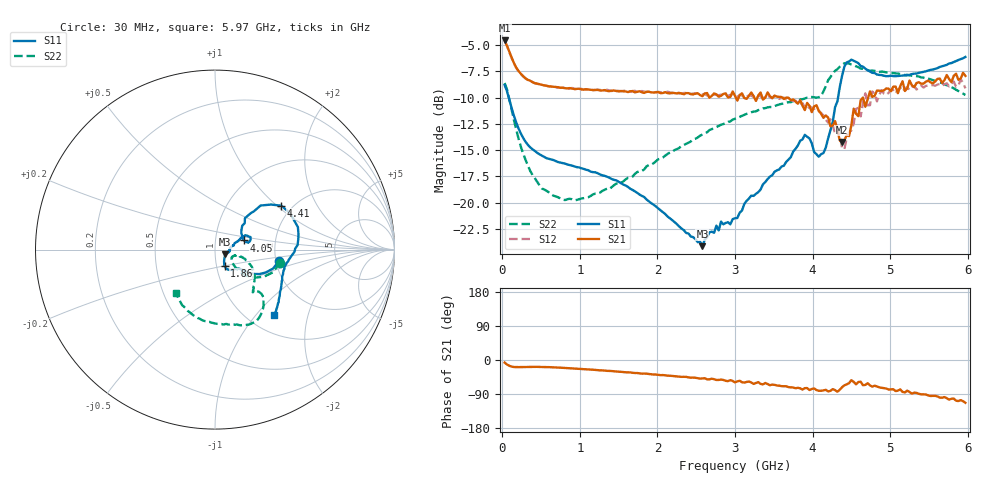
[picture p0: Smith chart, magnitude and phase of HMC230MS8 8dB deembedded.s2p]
!Hittite Microwave Corporation
!12 Elizabeth Drive
!Chelmsford, MA 01824
!Tel: 978-250-3343
!Fax: 978-250-3373
!Device: HMC230MS8, 0.75-2 GHz GaAs IC 3-bit Digital Attenuator in 8 lead plastic surface mount Mini Small Outline Package
!Misc: Room Temp Vdd = 5V , 8dB State.
# GHZ S DB R 50.0
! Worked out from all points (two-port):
!   199 points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, 30 MHz to 5.97 GHz, reference 50 ohm
!   highest |S21| = -4.57 dB at 30 MHz (marker M1); lowest = -14.2 dB at 4.38 GHz (marker M2)
!   |S21| within 3 dB of the highest: start of sweep to 220 MHz
!   lowest |S11| = -24.1 dB at 2.58 GHz (marker M3), VSWR 1.13, Z = 55.9 - j2.93 ohm
!   |S11| at or under -10 dB: 82.68 MHz to 4.328 GHz (4.246 GHz wide, 193 % of centre)
!   |S22| runs from -19.8 to -6.7 dB; largest |S21 - S12| = 0.057
!   S11 on the Smith chart (normalised r, x): 30 MHz: 2.08, -0.31; 1.86 GHz: 1.09, -0.20; 4.05 GHz: 1.38, +0.14; 4.41 GHz: 1.76, +1.07; 5.97 GHz: 1.30, -1.26
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0.03  -8.81 -10.2  -4.57 -6.8  -4.63 -6.6  -8.62 -11.2
0.18  -12.38 -33.4  -7.16 -18.7  -7.16 -18.8  -13.06 -39.9
0.39  -14.92 -37.4  -8.53 -18.3  -8.54 -18.1  -17.37 -39.6
1.02  -16.73 -50.9  -9.23 -23.8  -9.17 -23.7  -19.60 -21.9
1.86  -19.70 -58.9  -9.46 -36.2  -9.46 -36.4  -16.54 -15.6
2.04  -20.73 -56.6  -9.58 -39.9  -9.50 -39.6  -15.81 -15.8
2.58  -24.14 -24.9  -9.87 -48.6  -9.71 -48.9  -13.52 -22.8
3  -21.48 3.2  -9.83 -59.1  -9.86 -57.2  -12.02 -30.4
3.9  -13.55 19.4  -11.19 -74.2  -10.92 -78.4  -10.09 -47.4
3.99  -14.36 11.5  -11.39 -76.5  -10.95 -78.2  -9.95 -48.4
4.05  -15.39 17.5  -10.73 -79.3  -11.04 -79.4  -10.01 -47.9
4.17  -14.77 36.4  -11.70 -78.7  -12.11 -83.0  -8.93 -43.5
4.38  -7.94 38.8  -14.23 -71.8  -14.82 -78.1  -6.89 -57.1
4.41  -7.06 33.5  -14.06 -66.9  -14.92 -67.3  -6.74 -59.9
4.47  -6.57 20.6  -13.67 -61.1  -13.25 -62.5  -6.77 -65.3
4.53  -6.50 10.6  -11.06 -57.7  -12.50 -55.7  -6.93 -69.4
4.62  -7.00 0.7  -10.25 -57.2  -11.80 -62.8  -7.25 -73.7
4.68  -7.25 -3.4  -10.88 -65.8  -9.60 -67.0  -7.32 -75.7
4.71  -7.42 -5.2  -10.17 -61.4  -10.75 -71.5  -7.39 -77.1
4.77  -7.65 -8.0  -9.94 -70.2  -9.42 -66.7  -7.43 -79.2
4.98  -7.96 -14.9  -9.16 -78.0  -9.56 -76.2  -7.63 -86.1
5.97  -6.14 -47.9  -7.94 -113.0  -9.13 -110.5  -9.76 -132.4
